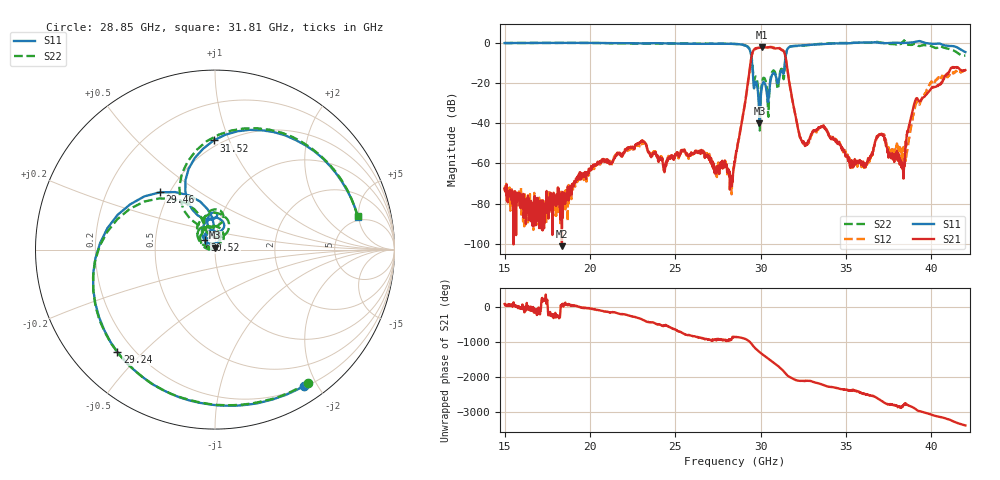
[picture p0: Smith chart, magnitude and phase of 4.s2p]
!The following data was pulled from an Agilent PNA
!This sNp file was generated from the data in the RF Test software
!NOTE:  Smoothing/Math/Corrections applied on any given trace ARE included in the data saved here
# MHz S dB R 50
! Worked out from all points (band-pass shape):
!   1601 points, 15 GHz to 42 GHz, reference 50 ohm
!   highest |S21| = -2.10 dB at 30.1 GHz (marker M1); lowest = -101.2 dB at 18.36 GHz (marker M2)
!   |S21| within 3 dB of the highest: 29.52 GHz to 31.4 GHz (1.885 GHz wide, 6.19 % of centre)
!   lowest |S11| = -40.0 dB at 29.93 GHz (marker M3), VSWR 1.02, Z = 49.9 + j0.989 ohm
!   |S11| at or under -10 dB: 29.5 GHz to 31.42 GHz (1.921 GHz wide, 6.31 % of centre)
!   |S22| runs from -43.7 to 1.1 dB; largest |S21 - S12| = 0.084
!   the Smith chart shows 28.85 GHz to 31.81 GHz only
!   S11 on the Smith chart (normalised r, x): 28.85 GHz: 0.21, -1.82; 29.24 GHz: 0.14, -0.42; 29.46 GHz: 0.44, +0.35; 30.52 GHz: 0.89, +0.09; 31.52 GHz: 0.45, +0.88; 31.81 GHz: 4.46, +4.87
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15000  -0.17 18.7  -72.69 96.0  -71.80 83.3  -0.14 17.7
18358.12  -0.06 -46.4  -101.20 93.4  -79.06 58.9  -0.09 -47.6
19505.62  -0.07 -72.5  -65.01 -3.1  -67.41 -1.2  -0.12 -73.8
24011.25  -0.24 158.4  -58.20 -131.4  -57.32 -127.8  -0.44 158.6
26559.38  -0.54 75.6  -54.97 -158.1  -53.97 -157.2  -0.42 76.2
28500  -0.62 -19.4  -59.25 -128.7  -57.46 -127.8  -0.61 -18.6
28854.38  -0.85 -57.0  -41.63 -148.9  -41.29 -151.4  -0.87 -55.1
29242.5  -2.06 -133.6  -20.57 138.5  -21.34 133.4  -1.93 -127.7
29461.88  -7.08 133.8  -7.19 38.5  -7.50 41.4  -6.44 145.8
29934.38  -40.00 97.5  -2.51 159.3  -2.51 159.8  -40.95 54.5
30103.12  -20.96 125.3  -2.10 93.8  -2.29 95.6  -18.87 135.5
30525  -22.38 136.9  -2.15 -58.1  -2.20 -57.0  -22.38 157.0
30828.75  -15.32 80.3  -2.81 -168.5  -2.53 -168.5  -14.39 73.4
31065  -18.64 102.2  -2.72 100.3  -2.58 101.0  -19.19 115.0
31520.62  -4.32 90.7  -10.51 -131.5  -10.10 -132.9  -4.36 94.5
31807.5  -1.76 12.9  -25.60 133.1  -26.17 132.9  -1.76 13.1
32330.62  -1.43 -91.5  -47.21 50.8  -47.12 52.4  -1.56 -93.0
33005.62  -0.99 176.4  -45.01 36.4  -45.53 35.9  -0.98 175.2
34490.62  -0.31 93.4  -49.09 -157.3  -49.48 -155.0  -0.16 91.3
37511.25  -0.14 26.6  -56.48 101.6  -53.68 105.5  -0.54 19.7
38304.38  -0.11 13.6  -62.61 56.4  -55.90 -1.1  -0.05 15.3
42000  -4.62 -66.0  -13.60 -147.3  -13.79 -140.0  -6.39 -42.0
